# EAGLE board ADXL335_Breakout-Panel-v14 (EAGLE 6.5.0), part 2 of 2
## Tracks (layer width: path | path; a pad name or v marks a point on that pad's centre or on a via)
GND  (via drill 0.51)
  Top 0.254: 19.05,16.26 18.8,16.51 | C2.2 18.29,9.56
  other vias: 13.59,17.02 13.21,19.56 16.89,17.91 17.5,7.82
  pour Bottom: 6.86,22.1 24.64,22.1 24.64,6.86 6.86,6.86
  pour Top: 6.86,6.86 24.64,6.86 24.64,22.1 6.86,22.1
GND1  (via drill 0.51)
  Top 0.254: 37.34,16.26 37.08,16.51 | C6.2 36.58,9.56
  other vias: 31.88,17.02 31.5,19.56 35.18,17.91 35.79,7.82
  pour Bottom: 25.15,22.1 42.93,22.1 42.93,6.86 25.15,6.86
  pour Top: 25.15,6.86 42.93,6.86 42.93,22.1 25.15,22.1
GND2  (via drill 0.51)
  Top 0.254: 55.63,16.26 55.37,16.51 | C10.2 54.86,9.56
  other vias: 50.16,17.02 49.78,19.56 53.47,17.91 54.08,7.82
  pour Bottom: 43.43,22.1 61.21,22.1 61.21,6.86 43.43,6.86
  pour Top: 43.43,6.86 61.21,6.86 61.21,22.1 43.43,22.1
GND3  (via drill 0.51)
  Top 0.254: 73.91,16.26 73.66,16.51 | C14.2 73.15,9.56
  other vias: 68.45,17.02 68.07,19.56 71.75,17.91 72.36,7.82
  pour Bottom: 61.72,22.1 79.5,22.1 79.5,6.86 61.72,6.86
  pour Top: 61.72,6.86 79.5,6.86 79.5,22.1 61.72,22.1
GND4  (via drill 0.51)
  Top 0.254: 92.2,16.26 91.95,16.51 | C18.2 91.44,9.56
  other vias: 86.74,17.02 86.36,19.56 90.04,17.91 90.65,7.82
  pour Bottom: 80.01,22.1 97.79,22.1 97.79,6.86 80.01,6.86
  pour Top: 80.01,6.86 97.79,6.86 97.79,22.1 80.01,22.1
GND5  (via drill 0.51)
  Top 0.254: 110.49,16.26 110.24,16.51 | C22.2 109.73,9.56
  other vias: 105.03,17.02 104.65,19.56 108.33,17.91 108.94,7.82
  pour Bottom: 98.3,22.1 116.08,22.1 116.08,6.86 98.3,6.86
  pour Top: 98.3,6.86 116.08,6.86 116.08,22.1 98.3,22.1
GND6  (via drill 0.51)
  Top 0.254: 19.05,32 18.8,32.26 | C26.2 18.29,25.31
  other vias: 13.59,32.77 13.21,35.31 16.89,33.66 17.5,23.57
  pour Bottom: 6.86,37.85 24.64,37.85 24.64,22.61 6.86,22.61
  pour Top: 6.86,22.61 24.64,22.61 24.64,37.85 6.86,37.85
GND7  (via drill 0.51)
  Top 0.254: 37.34,32 37.08,32.26 | C30.2 36.58,25.31
  other vias: 31.88,32.77 31.5,35.31 35.18,33.66 35.79,23.57
  pour Bottom: 25.15,37.85 42.93,37.85 42.93,22.61 25.15,22.61
  pour Top: 25.15,22.61 42.93,22.61 42.93,37.85 25.15,37.85
GND8  (via drill 0.51)
  Top 0.254: 55.63,32 55.37,32.26 | C34.2 54.86,25.31
  other vias: 50.16,32.77 49.78,35.31 53.47,33.66 54.08,23.57
  pour Bottom: 43.43,37.85 61.21,37.85 61.21,22.61 43.43,22.61
  pour Top: 43.43,22.61 61.21,22.61 61.21,37.85 43.43,37.85
GND9  (via drill 0.51)
  Top 0.254: 73.91,32 73.66,32.26 | C38.2 73.15,25.31
  other vias: 68.45,32.77 68.07,35.31 71.75,33.66 72.36,23.57
  pour Bottom: 61.72,37.85 79.5,37.85 79.5,22.61 61.72,22.61
  pour Top: 61.72,22.61 79.5,22.61 79.5,37.85 61.72,37.85
GND10  (via drill 0.51)
  Top 0.254: 92.2,32 91.95,32.26 | C42.2 91.44,25.31
  other vias: 86.74,32.77 86.36,35.31 90.04,33.66 90.65,23.57
  pour Bottom: 80.01,37.85 97.79,37.85 97.79,22.61 80.01,22.61
  pour Top: 80.01,22.61 97.79,22.61 97.79,37.85 80.01,37.85
GND11  (via drill 0.51)
  Top 0.254: 110.49,32 110.24,32.26 | C46.2 109.73,25.31
  other vias: 105.03,32.77 104.65,35.31 108.33,33.66 108.94,23.57
  pour Bottom: 98.3,37.85 116.08,37.85 116.08,22.61 98.3,22.61
  pour Top: 98.3,22.61 116.08,22.61 116.08,37.85 98.3,37.85
GND12  (via drill 0.51)
  Top 0.254: 19.05,47.75 18.8,48.01 | C50.2 18.29,41.06
  other vias: 13.59,48.51 13.21,51.05 16.89,49.4 17.5,39.32
  pour Bottom: 6.86,53.59 24.64,53.59 24.64,38.35 6.86,38.35
  pour Top: 6.86,38.35 24.64,38.35 24.64,53.59 6.86,53.59
GND13  (via drill 0.51)
  Top 0.254: 37.34,47.75 37.08,48.01 | C54.2 36.58,41.06
  other vias: 31.88,48.51 31.5,51.05 35.18,49.4 35.79,39.32
  pour Bottom: 25.15,53.59 42.93,53.59 42.93,38.35 25.15,38.35
  pour Top: 25.15,38.35 42.93,38.35 42.93,53.59 25.15,53.59
GND14  (via drill 0.51)
  Top 0.254: 55.63,47.75 55.37,48.01 | C58.2 54.86,41.06
  other vias: 50.16,48.51 49.78,51.05 53.47,49.4 54.08,39.32
  pour Bottom: 43.43,53.59 61.21,53.59 61.21,38.35 43.43,38.35
  pour Top: 43.43,38.35 61.21,38.35 61.21,53.59 43.43,53.59
GND15  (via drill 0.51)
  Top 0.254: 73.91,47.75 73.66,48.01 | C62.2 73.15,41.06
  other vias: 68.45,48.51 68.07,51.05 71.75,49.4 72.36,39.32
  pour Bottom: 61.72,53.59 79.5,53.59 79.5,38.35 61.72,38.35
  pour Top: 61.72,38.35 79.5,38.35 79.5,53.59 61.72,53.59
GND16  (via drill 0.51)
  Top 0.254: 92.2,47.75 91.95,48.01 | C66.2 91.44,41.06
  other vias: 86.74,48.51 86.36,51.05 90.04,49.4 90.65,39.32
  pour Bottom: 80.01,53.59 97.79,53.59 97.79,38.35 80.01,38.35
  pour Top: 80.01,38.35 97.79,38.35 97.79,53.59 80.01,53.59
GND17  (via drill 0.51)
  Top 0.254: 110.49,47.75 110.24,48.01 | C70.2 109.73,41.06
  other vias: 105.03,48.51 104.65,51.05 108.33,49.4 108.94,39.32
  pour Bottom: 98.3,53.59 116.08,53.59 116.08,38.35 98.3,38.35
  pour Top: 98.3,38.35 116.08,38.35 116.08,53.59 98.3,53.59
GND18  (via drill 0.51)
  Top 0.254: 19.05,63.5 18.8,63.75 | C74.2 18.29,56.81
  other vias: 13.59,64.26 13.21,66.8 16.89,65.15 17.5,55.07
  pour Bottom: 6.86,69.34 24.64,69.34 24.64,54.1 6.86,54.1
  pour Top: 6.86,54.1 24.64,54.1 24.64,69.34 6.86,69.34
GND19  (via drill 0.51)
  Top 0.254: 37.34,63.5 37.08,63.75 | C78.2 36.58,56.81
  other vias: 31.88,64.26 31.5,66.8 35.18,65.15 35.79,55.07
  pour Bottom: 25.15,69.34 42.93,69.34 42.93,54.1 25.15,54.1
  pour Top: 25.15,54.1 42.93,54.1 42.93,69.34 25.15,69.34
GND20  (via drill 0.51)
  Top 0.254: 55.63,63.5 55.37,63.75 | C82.2 54.86,56.81
  other vias: 50.16,64.26 49.78,66.8 53.47,65.15 54.08,55.07
  pour Bottom: 43.43,69.34 61.21,69.34 61.21,54.1 43.43,54.1
  pour Top: 43.43,54.1 61.21,54.1 61.21,69.34 43.43,69.34
GND21  (via drill 0.51)
  Top 0.254: 73.91,63.5 73.66,63.75 | C86.2 73.15,56.81
  other vias: 68.45,64.26 68.07,66.8 71.75,65.15 72.36,55.07
  pour Bottom: 61.72,69.34 79.5,69.34 79.5,54.1 61.72,54.1
  pour Top: 61.72,54.1 79.5,54.1 79.5,69.34 61.72,69.34
GND22  (via drill 0.51)
  Top 0.254: 92.2,63.5 91.95,63.75 | C90.2 91.44,56.81
  other vias: 86.74,64.26 86.36,66.8 90.04,65.15 90.65,55.07
  pour Bottom: 80.01,69.34 97.79,69.34 97.79,54.1 80.01,54.1
  pour Top: 80.01,54.1 97.79,54.1 97.79,69.34 80.01,69.34
GND23  (via drill 0.51)
  Top 0.254: 110.49,63.5 110.24,63.75 | C94.2 109.73,56.81
  other vias: 105.03,64.26 104.65,66.8 108.33,65.15 108.94,55.07
  pour Bottom: 98.3,69.34 116.08,69.34 116.08,54.1 98.3,54.1
  pour Top: 98.3,54.1 116.08,54.1 116.08,69.34 98.3,69.34
GND24  (via drill 0.51)
  Top 0.254: 19.05,79.25 18.8,79.5 | C98.2 18.29,72.56
  other vias: 13.59,80.01 13.21,82.55 16.89,80.9 17.5,70.82
  pour Bottom: 6.86,85.09 24.64,85.09 24.64,69.85 6.86,69.85
  pour Top: 6.86,69.85 24.64,69.85 24.64,85.09 6.86,85.09
GND25  (via drill 0.51)
  Top 0.254: 37.34,79.25 37.08,79.5 | C102.2 36.58,72.56
  other vias: 31.88,80.01 31.5,82.55 35.18,80.9 35.79,70.82
  pour Bottom: 25.15,85.09 42.93,85.09 42.93,69.85 25.15,69.85
  pour Top: 25.15,69.85 42.93,69.85 42.93,85.09 25.15,85.09
GND26  (via drill 0.51)
  Top 0.254: 55.63,79.25 55.37,79.5 | C106.2 54.86,72.56
  other vias: 50.16,80.01 49.78,82.55 53.47,80.9 54.08,70.82
  pour Bottom: 43.43,85.09 61.21,85.09 61.21,69.85 43.43,69.85
  pour Top: 43.43,69.85 61.21,69.85 61.21,85.09 43.43,85.09
GND27  (via drill 0.51)
  Top 0.254: 73.91,79.25 73.66,79.5 | C110.2 73.15,72.56
  other vias: 68.45,80.01 68.07,82.55 71.75,80.9 72.36,70.82
  pour Bottom: 61.72,85.09 79.5,85.09 79.5,69.85 61.72,69.85
  pour Top: 61.72,69.85 79.5,69.85 79.5,85.09 61.72,85.09
GND28  (via drill 0.51)
  Top 0.254: 92.2,79.25 91.95,79.5 | C114.2 91.44,72.56
  other vias: 86.74,80.01 86.36,82.55 90.04,80.9 90.65,70.82
  pour Bottom: 80.01,85.09 97.79,85.09 97.79,69.85 80.01,69.85
  pour Top: 80.01,69.85 97.79,69.85 97.79,85.09 80.01,85.09
GND29  (via drill 0.51)
  Top 0.254: 110.49,79.25 110.24,79.5 | C118.2 109.73,72.56
  other vias: 105.03,80.01 104.65,82.55 108.33,80.9 108.94,70.82
  pour Bottom: 98.3,85.09 116.08,85.09 116.08,69.85 98.3,69.85
  pour Top: 98.3,69.85 116.08,69.85 116.08,85.09 98.3,85.09
GND30  (via drill 0.51)
  Top 0.254: 19.05,95 18.8,95.25 | C122.2 18.29,88.3
  other vias: 13.59,95.76 13.21,98.3 16.89,96.65 17.5,86.56
  pour Bottom: 6.86,100.84 24.64,100.84 24.64,85.6 6.86,85.6
  pour Top: 6.86,85.6 24.64,85.6 24.64,100.84 6.86,100.84
GND31  (via drill 0.51)
  Top 0.254: 37.34,95 37.08,95.25 | C126.2 36.58,88.3
  other vias: 31.88,95.76 31.5,98.3 35.18,96.65 35.79,86.56
  pour Bottom: 25.15,100.84 42.93,100.84 42.93,85.6 25.15,85.6
  pour Top: 25.15,85.6 42.93,85.6 42.93,100.84 25.15,100.84
GND32  (via drill 0.51)
  Top 0.254: 55.63,95 55.37,95.25 | C130.2 54.86,88.3
  other vias: 50.16,95.76 49.78,98.3 53.47,96.65 54.08,86.56
  pour Bottom: 43.43,100.84 61.21,100.84 61.21,85.6 43.43,85.6
  pour Top: 43.43,85.6 61.21,85.6 61.21,100.84 43.43,100.84
GND33  (via drill 0.51)
  Top 0.254: 73.91,95 73.66,95.25 | C134.2 73.15,88.3
  other vias: 68.45,95.76 68.07,98.3 71.75,96.65 72.36,86.56
  pour Bottom: 61.72,100.84 79.5,100.84 79.5,85.6 61.72,85.6
  pour Top: 61.72,85.6 79.5,85.6 79.5,100.84 61.72,100.84
GND34  (via drill 0.51)
  Top 0.254: 92.2,95 91.95,95.25 | C138.2 91.44,88.3
  other vias: 86.74,95.76 86.36,98.3 90.04,96.65 90.65,86.56
  pour Bottom: 80.01,100.84 97.79,100.84 97.79,85.6 80.01,85.6
  pour Top: 80.01,85.6 97.79,85.6 97.79,100.84 80.01,100.84
GND35  (via drill 0.51)
  Top 0.254: 110.49,95 110.24,95.25 | C142.2 109.73,88.3
  other vias: 105.03,95.76 104.65,98.3 108.33,96.65 108.94,86.56
  pour Bottom: 98.3,100.84 116.08,100.84 116.08,85.6 98.3,85.6
  pour Top: 98.3,85.6 116.08,85.6 116.08,100.84 98.3,100.84
GND36  (via drill 0.51)
  Top 0.254: 19.05,110.74 18.8,111 | C146.2 18.29,104.05
  other vias: 13.59,111.51 13.21,114.05 16.89,112.39 17.5,102.31
  pour Bottom: 6.86,116.59 24.64,116.59 24.64,101.35 6.86,101.35
  pour Top: 6.86,101.35 24.64,101.35 24.64,116.59 6.86,116.59
GND37  (via drill 0.51)
  Top 0.254: 37.34,110.74 37.08,111 | C150.2 36.58,104.05
  other vias: 31.88,111.51 31.5,114.05 35.18,112.39 35.79,102.31
  pour Bottom: 25.15,116.59 42.93,116.59 42.93,101.35 25.15,101.35
  pour Top: 25.15,101.35 42.93,101.35 42.93,116.59 25.15,116.59
GND38  (via drill 0.51)
  Top 0.254: 55.63,110.74 55.37,111 | C154.2 54.86,104.05
  other vias: 50.16,111.51 49.78,114.05 53.47,112.39 54.08,102.31
  pour Bottom: 43.43,116.59 61.21,116.59 61.21,101.35 43.43,101.35
  pour Top: 43.43,101.35 61.21,101.35 61.21,116.59 43.43,116.59
GND39  (via drill 0.51)
  Top 0.254: 73.91,110.74 73.66,111 | C158.2 73.15,104.05
  other vias: 68.45,111.51 68.07,114.05 71.75,112.39 72.36,102.31
  pour Bottom: 61.72,116.59 79.5,116.59 79.5,101.35 61.72,101.35
  pour Top: 61.72,101.35 79.5,101.35 79.5,116.59 61.72,116.59
GND40  (via drill 0.51)
  Top 0.254: 92.2,110.74 91.95,111 | C162.2 91.44,104.05
  other vias: 86.74,111.51 86.36,114.05 90.04,112.39 90.65,102.31
  pour Bottom: 80.01,116.59 97.79,116.59 97.79,101.35 80.01,101.35
  pour Top: 80.01,101.35 97.79,101.35 97.79,116.59 80.01,116.59
GND41  (via drill 0.51)
  Top 0.254: 110.49,110.74 110.24,111 | C166.2 109.73,104.05
  other vias: 105.03,111.51 104.65,114.05 108.33,112.39 108.94,102.31
  pour Bottom: 98.3,116.59 116.08,116.59 116.08,101.35 98.3,101.35
  pour Top: 98.3,101.35 116.08,101.35 116.08,116.59 98.3,116.59
ST  (via drill 0.51)
  Top 0.254: U$4.2 18.39,14.1 v20.95,14.1
  Bottom 0.254: v20.95,14.1 13.59,14.1 11.94,15.75 11.94,19.56 10.67,20.83 SL1.1
ST1  (via drill 0.51)
  Top 0.254: U$10.2 36.68,14.1 v39.24,14.1
  Bottom 0.254: v39.24,14.1 31.88,14.1 30.23,15.75 30.23,19.56 28.96,20.83 SL2.1
ST2  (via drill 0.51)
  Top 0.254: U$17.2 54.97,14.1 v57.53,14.1
  Bottom 0.254: v57.53,14.1 50.16,14.1 48.51,15.75 48.51,19.56 47.24,20.83 SL3.1
ST3  (via drill 0.51)
  Top 0.254: U$24.2 73.26,14.1 v75.82,14.1
  Bottom 0.254: v75.82,14.1 68.45,14.1 66.8,15.75 66.8,19.56 65.53,20.83 SL4.1
ST4  (via drill 0.51)
  Top 0.254: U$31.2 91.54,14.1 v94.11,14.1
  Bottom 0.254: v94.11,14.1 86.74,14.1 85.09,15.75 85.09,19.56 83.82,20.83 SL5.1
ST5  (via drill 0.51)
  Top 0.254: U$38.2 109.83,14.1 v112.39,14.1
  Bottom 0.254: v112.39,14.1 105.03,14.1 103.38,15.75 103.38,19.56 102.11,20.83 SL6.1
ST6  (via drill 0.51)
  Top 0.254: U$45.2 18.39,29.84 v20.95,29.84
  Bottom 0.254: v20.95,29.84 13.59,29.84 11.94,31.5 11.94,35.31 10.67,36.58 SL7.1
ST7  (via drill 0.51)
  Top 0.254: U$52.2 36.68,29.84 v39.24,29.84
  Bottom 0.254: v39.24,29.84 31.88,29.84 30.23,31.5 30.23,35.31 28.96,36.58 SL8.1
ST8  (via drill 0.51)
  Top 0.254: U$59.2 54.97,29.84 v57.53,29.84
  Bottom 0.254: v57.53,29.84 50.16,29.84 48.51,31.5 48.51,35.31 47.24,36.58 SL9.1
ST9  (via drill 0.51)
  Top 0.254: U$66.2 73.26,29.84 v75.82,29.84
  Bottom 0.254: v75.82,29.84 68.45,29.84 66.8,31.5 66.8,35.31 65.53,36.58 SL10.1
ST10  (via drill 0.51)
  Top 0.254: U$73.2 91.54,29.84 v94.11,29.84
  Bottom 0.254: v94.11,29.84 86.74,29.84 85.09,31.5 85.09,35.31 83.82,36.58 SL11.1
ST11  (via drill 0.51)
  Top 0.254: U$80.2 109.83,29.84 v112.39,29.84
  Bottom 0.254: v112.39,29.84 105.03,29.84 103.38,31.5 103.38,35.31 102.11,36.58 SL12.1
ST12  (via drill 0.51)
  Top 0.254: U$87.2 18.39,45.59 v20.95,45.59
  Bottom 0.254: v20.95,45.59 13.59,45.59 11.94,47.24 11.94,51.05 10.67,52.32 SL13.1
ST13  (via drill 0.51)
  Top 0.254: U$94.2 36.68,45.59 v39.24,45.59
  Bottom 0.254: v39.24,45.59 31.88,45.59 30.23,47.24 30.23,51.05 28.96,52.32 SL14.1
ST14  (via drill 0.51)
  Top 0.254: U$101.2 54.97,45.59 v57.53,45.59
  Bottom 0.254: v57.53,45.59 50.16,45.59 48.51,47.24 48.51,51.05 47.24,52.32 SL15.1
ST15  (via drill 0.51)
  Top 0.254: U$108.2 73.26,45.59 v75.82,45.59
  Bottom 0.254: v75.82,45.59 68.45,45.59 66.8,47.24 66.8,51.05 65.53,52.32 SL16.1
ST16  (via drill 0.51)
  Top 0.254: U$115.2 91.54,45.59 v94.11,45.59
  Bottom 0.254: v94.11,45.59 86.74,45.59 85.09,47.24 85.09,51.05 83.82,52.32 SL17.1
ST17  (via drill 0.51)
  Top 0.254: U$122.2 109.83,45.59 v112.39,45.59
  Bottom 0.254: v112.39,45.59 105.03,45.59 103.38,47.24 103.38,51.05 102.11,52.32 SL18.1
ST18  (via drill 0.51)
  Top 0.254: U$129.2 18.39,61.34 v20.95,61.34
  Bottom 0.254: v20.95,61.34 13.59,61.34 11.94,62.99 11.94,66.8 10.67,68.07 SL19.1
ST19  (via drill 0.51)
  Top 0.254: U$136.2 36.68,61.34 v39.24,61.34
  Bottom 0.254: v39.24,61.34 31.88,61.34 30.23,62.99 30.23,66.8 28.96,68.07 SL20.1
ST20  (via drill 0.51)
  Top 0.254: U$143.2 54.97,61.34 v57.53,61.34
  Bottom 0.254: v57.53,61.34 50.16,61.34 48.51,62.99 48.51,66.8 47.24,68.07 SL21.1
ST21  (via drill 0.51)
  Top 0.254: U$150.2 73.26,61.34 v75.82,61.34
  Bottom 0.254: v75.82,61.34 68.45,61.34 66.8,62.99 66.8,66.8 65.53,68.07 SL22.1
ST22  (via drill 0.51)
  Top 0.254: U$157.2 91.54,61.34 v94.11,61.34
  Bottom 0.254: v94.11,61.34 86.74,61.34 85.09,62.99 85.09,66.8 83.82,68.07 SL23.1
ST23  (via drill 0.51)
  Top 0.254: U$164.2 109.83,61.34 v112.39,61.34
  Bottom 0.254: v112.39,61.34 105.03,61.34 103.38,62.99 103.38,66.8 102.11,68.07 SL24.1
ST24  (via drill 0.51)
  Top 0.254: U$171.2 18.39,77.09 v20.95,77.09
  Bottom 0.254: v20.95,77.09 13.59,77.09 11.94,78.74 11.94,82.55 10.67,83.82 SL25.1
ST25  (via drill 0.51)
  Top 0.254: U$178.2 36.68,77.09 v39.24,77.09
  Bottom 0.254: v39.24,77.09 31.88,77.09 30.23,78.74 30.23,82.55 28.96,83.82 SL26.1
ST26  (via drill 0.51)
  Top 0.254: U$185.2 54.97,77.09 v57.53,77.09
  Bottom 0.254: v57.53,77.09 50.16,77.09 48.51,78.74 48.51,82.55 47.24,83.82 SL27.1
ST27  (via drill 0.51)
  Top 0.254: U$192.2 73.26,77.09 v75.82,77.09
  Bottom 0.254: v75.82,77.09 68.45,77.09 66.8,78.74 66.8,82.55 65.53,83.82 SL28.1
ST28  (via drill 0.51)
  Top 0.254: U$199.2 91.54,77.09 v94.11,77.09
  Bottom 0.254: v94.11,77.09 86.74,77.09 85.09,78.74 85.09,82.55 83.82,83.82 SL29.1
ST29  (via drill 0.51)
  Top 0.254: U$206.2 109.83,77.09 v112.39,77.09
  Bottom 0.254: v112.39,77.09 105.03,77.09 103.38,78.74 103.38,82.55 102.11,83.82 SL30.1
ST30  (via drill 0.51)
  Top 0.254: U$213.2 18.39,92.84 v20.95,92.84
  Bottom 0.254: v20.95,92.84 13.59,92.84 11.94,94.49 11.94,98.3 10.67,99.57 SL31.1
ST31  (via drill 0.51)
  Top 0.254: U$220.2 36.68,92.84 v39.24,92.84
  Bottom 0.254: v39.24,92.84 31.88,92.84 30.23,94.49 30.23,98.3 28.96,99.57 SL32.1
ST32  (via drill 0.51)
  Top 0.254: U$227.2 54.97,92.84 v57.53,92.84
  Bottom 0.254: v57.53,92.84 50.16,92.84 48.51,94.49 48.51,98.3 47.24,99.57 SL33.1
ST33  (via drill 0.51)
  Top 0.254: U$234.2 73.26,92.84 v75.82,92.84
  Bottom 0.254: v75.82,92.84 68.45,92.84 66.8,94.49 66.8,98.3 65.53,99.57 SL34.1
ST34  (via drill 0.51)
  Top 0.254: U$241.2 91.54,92.84 v94.11,92.84
  Bottom 0.254: v94.11,92.84 86.74,92.84 85.09,94.49 85.09,98.3 83.82,99.57 SL35.1
ST35  (via drill 0.51)
  Top 0.254: U$248.2 109.83,92.84 v112.39,92.84
  Bottom 0.254: v112.39,92.84 105.03,92.84 103.38,94.49 103.38,98.3 102.11,99.57 SL36.1
ST36  (via drill 0.51)
  Top 0.254: U$255.2 18.39,108.58 v20.95,108.58
  Bottom 0.254: v20.95,108.58 13.59,108.58 11.94,110.24 11.94,114.05 10.67,115.32 SL37.1
ST37  (via drill 0.51)
  Top 0.254: U$262.2 36.68,108.58 v39.24,108.58
  Bottom 0.254: v39.24,108.58 31.88,108.58 30.23,110.24 30.23,114.05 28.96,115.32 SL38.1
ST38  (via drill 0.51)
  Top 0.254: U$269.2 54.97,108.58 v57.53,108.58
  Bottom 0.254: v57.53,108.58 50.16,108.58 48.51,110.24 48.51,114.05 47.24,115.32 SL39.1
ST39  (via drill 0.51)
  Top 0.254: U$276.2 73.26,108.58 v75.82,108.58
  Bottom 0.254: v75.82,108.58 68.45,108.58 66.8,110.24 66.8,114.05 65.53,115.32 SL40.1
ST40  (via drill 0.51)
  Top 0.254: U$283.2 91.54,108.58 v94.11,108.58
  Bottom 0.254: v94.11,108.58 86.74,108.58 85.09,110.24 85.09,114.05 83.82,115.32 SL41.1
ST41  (via drill 0.51)
  Top 0.254: U$290.2 109.83,108.58 v112.39,108.58
  Bottom 0.254: v112.39,108.58 105.03,108.58 103.38,110.24 103.38,114.05 102.11,115.32 SL42.1
VCC
  Top 0.254: U$4.14 16.18,11.63 16.51,11.3 | U$4.15 16.84,11.63 16.51,11.3 | SL1.6 15.15,8.13 C2.1 16.51,9.56 16.51,11.3
VCC1
  Top 0.254: U$10.14 34.47,11.63 34.8,11.3 | U$10.15 35.12,11.63 34.8,11.3 | SL2.6 33.44,8.13 C6.1 34.8,9.56 34.8,11.3
VCC2
  Top 0.254: U$17.14 52.76,11.63 53.09,11.3 | U$17.15 53.41,11.63 53.09,11.3 | SL3.6 51.73,8.13 C10.1 53.09,9.56 53.09,11.3
VCC3
  Top 0.254: U$24.14 71.05,11.63 71.37,11.3 | U$24.15 71.7,11.63 71.37,11.3 | SL4.6 70.02,8.13 C14.1 71.37,9.56 71.37,11.3
VCC4
  Top 0.254: U$31.14 89.34,11.63 89.66,11.3 | U$31.15 89.99,11.63 89.66,11.3 | SL5.6 88.3,8.13 C18.1 89.66,9.56 89.66,11.3
VCC5
  Top 0.254: U$38.14 107.62,11.63 107.95,11.3 | U$38.15 108.28,11.63 107.95,11.3 | SL6.6 106.59,8.13 C22.1 107.95,9.56 107.95,11.3
VCC6
  Top 0.254: U$45.14 16.18,27.38 16.51,27.05 | U$45.15 16.84,27.38 16.51,27.05 | SL7.6 15.15,23.88 C26.1 16.51,25.31 16.51,27.05
VCC7
  Top 0.254: U$52.14 34.47,27.38 34.8,27.05 | U$52.15 35.12,27.38 34.8,27.05 | SL8.6 33.44,23.88 C30.1 34.8,25.31 34.8,27.05
VCC8
  Top 0.254: U$59.14 52.76,27.38 53.09,27.05 | U$59.15 53.41,27.38 53.09,27.05 | SL9.6 51.73,23.88 C34.1 53.09,25.31 53.09,27.05
VCC9
  Top 0.254: U$66.14 71.05,27.38 71.37,27.05 | U$66.15 71.7,27.38 71.37,27.05 | SL10.6 70.02,23.88 C38.1 71.37,25.31 71.37,27.05
VCC10
  Top 0.254: U$73.14 89.34,27.38 89.66,27.05 | U$73.15 89.99,27.38 89.66,27.05 | SL11.6 88.3,23.88 C42.1 89.66,25.31 89.66,27.05
VCC11
  Top 0.254: U$80.14 107.62,27.38 107.95,27.05 | U$80.15 108.28,27.38 107.95,27.05 | SL12.6 106.59,23.88 C46.1 107.95,25.31 107.95,27.05
VCC12
  Top 0.254: U$87.14 16.18,43.12 16.51,42.8 | U$87.15 16.84,43.12 16.51,42.8 | SL13.6 15.15,39.62 C50.1 16.51,41.06 16.51,42.8
VCC13
  Top 0.254: U$94.14 34.47,43.12 34.8,42.8 | U$94.15 35.12,43.12 34.8,42.8 | SL14.6 33.44,39.62 C54.1 34.8,41.06 34.8,42.8
VCC14
  Top 0.254: U$101.14 52.76,43.12 53.09,42.8 | U$101.15 53.41,43.12 53.09,42.8 | SL15.6 51.73,39.62 C58.1 53.09,41.06 53.09,42.8
VCC15
  Top 0.254: U$108.14 71.05,43.12 71.37,42.8 | U$108.15 71.7,43.12 71.37,42.8 | SL16.6 70.02,39.62 C62.1 71.37,41.06 71.37,42.8
VCC16
  Top 0.254: U$115.14 89.34,43.12 89.66,42.8 | U$115.15 89.99,43.12 89.66,42.8 | SL17.6 88.3,39.62 C66.1 89.66,41.06 89.66,42.8
VCC17
  Top 0.254: U$122.14 107.62,43.12 107.95,42.8 | U$122.15 108.28,43.12 107.95,42.8 | SL18.6 106.59,39.62 C70.1 107.95,41.06 107.95,42.8
VCC18
  Top 0.254: U$129.14 16.18,58.87 16.51,58.55 | U$129.15 16.84,58.87 16.51,58.55 | SL19.6 15.15,55.37 C74.1 16.51,56.81 16.51,58.55
VCC19
  Top 0.254: U$136.14 34.47,58.87 34.8,58.55 | U$136.15 35.12,58.87 34.8,58.55 | SL20.6 33.44,55.37 C78.1 34.8,56.81 34.8,58.55
VCC20
  Top 0.254: U$143.14 52.76,58.87 53.09,58.55 | U$143.15 53.41,58.87 53.09,58.55 | SL21.6 51.73,55.37 C82.1 53.09,56.81 53.09,58.55
VCC21
  Top 0.254: U$150.14 71.05,58.87 71.37,58.55 | U$150.15 71.7,58.87 71.37,58.55 | SL22.6 70.02,55.37 C86.1 71.37,56.81 71.37,58.55
VCC22
  Top 0.254: U$157.14 89.34,58.87 89.66,58.55 | U$157.15 89.99,58.87 89.66,58.55 | SL23.6 88.3,55.37 C90.1 89.66,56.81 89.66,58.55
VCC23
  Top 0.254: U$164.14 107.62,58.87 107.95,58.55 | U$164.15 108.28,58.87 107.95,58.55 | SL24.6 106.59,55.37 C94.1 107.95,56.81 107.95,58.55
VCC24
  Top 0.254: U$171.14 16.18,74.62 16.51,74.3 | U$171.15 16.84,74.62 16.51,74.3 | SL25.6 15.15,71.12 C98.1 16.51,72.56 16.51,74.3
VCC25
  Top 0.254: U$178.14 34.47,74.62 34.8,74.3 | U$178.15 35.12,74.62 34.8,74.3 | SL26.6 33.44,71.12 C102.1 34.8,72.56 34.8,74.3
VCC26
  Top 0.254: U$185.14 52.76,74.62 53.09,74.3 | U$185.15 53.41,74.62 53.09,74.3 | SL27.6 51.73,71.12 C106.1 53.09,72.56 53.09,74.3
VCC27
  Top 0.254: U$192.14 71.05,74.62 71.37,74.3 | U$192.15 71.7,74.62 71.37,74.3 | SL28.6 70.02,71.12 C110.1 71.37,72.56 71.37,74.3
VCC28
  Top 0.254: U$199.14 89.34,74.62 89.66,74.3 | U$199.15 89.99,74.62 89.66,74.3 | SL29.6 88.3,71.12 C114.1 89.66,72.56 89.66,74.3
VCC29
  Top 0.254: U$206.14 107.62,74.62 107.95,74.3 | U$206.15 108.28,74.62 107.95,74.3 | SL30.6 106.59,71.12 C118.1 107.95,72.56 107.95,74.3
VCC30
  Top 0.254: U$213.14 16.18,90.37 16.51,90.04 | U$213.15 16.84,90.37 16.51,90.04 | SL31.6 15.15,86.87 C122.1 16.51,88.3 16.51,90.04
VCC31
  Top 0.254: U$220.14 34.47,90.37 34.8,90.04 | U$220.15 35.12,90.37 34.8,90.04 | SL32.6 33.44,86.87 C126.1 34.8,88.3 34.8,90.04
VCC32
  Top 0.254: U$227.14 52.76,90.37 53.09,90.04 | U$227.15 53.41,90.37 53.09,90.04 | SL33.6 51.73,86.87 C130.1 53.09,88.3 53.09,90.04
VCC33
  Top 0.254: U$234.14 71.05,90.37 71.37,90.04 | U$234.15 71.7,90.37 71.37,90.04 | SL34.6 70.02,86.87 C134.1 71.37,88.3 71.37,90.04
VCC34
  Top 0.254: U$241.14 89.34,90.37 89.66,90.04 | U$241.15 89.99,90.37 89.66,90.04 | SL35.6 88.3,86.87 C138.1 89.66,88.3 89.66,90.04
VCC35
  Top 0.254: U$248.14 107.62,90.37 107.95,90.04 | U$248.15 108.28,90.37 107.95,90.04 | SL36.6 106.59,86.87 C142.1 107.95,88.3 107.95,90.04
VCC36
  Top 0.254: U$255.14 16.18,106.12 16.51,105.79 | U$255.15 16.84,106.12 16.51,105.79 | SL37.6 15.15,102.62 C146.1 16.51,104.05 16.51,105.79
VCC37
  Top 0.254: U$262.14 34.47,106.12 34.8,105.79 | U$262.15 35.12,106.12 34.8,105.79 | SL38.6 33.44,102.62 C150.1 34.8,104.05 34.8,105.79
VCC38
  Top 0.254: U$269.14 52.76,106.12 53.09,105.79 | U$269.15 53.41,106.12 53.09,105.79 | SL39.6 51.73,102.62 C154.1 53.09,104.05 53.09,105.79
VCC39
  Top 0.254: U$276.14 71.05,106.12 71.37,105.79 | U$276.15 71.7,106.12 71.37,105.79 | SL40.6 70.02,102.62 C158.1 71.37,104.05 71.37,105.79
VCC40
  Top 0.254: U$283.14 89.34,106.12 89.66,105.79 | U$283.15 89.99,106.12 89.66,105.79 | SL41.6 88.3,102.62 C162.1 89.66,104.05 89.66,105.79
VCC41
  Top 0.254: U$290.14 107.62,106.12 107.95,105.79 | U$290.15 108.28,106.12 107.95,105.79 | SL42.6 106.59,102.62 C166.1 107.95,104.05 107.95,105.79
XOUT
  Top 0.254: U$4.12 12.24,13.5 C4.1 12.03,13.72 10.03,13.72 9.53,13.21 SL1.4
XOUT1
  Top 0.254: U$10.12 30.53,13.5 C8.1 30.31,13.72 28.32,13.72 27.81,13.21 SL2.4
XOUT2
  Top 0.254: U$17.12 48.81,13.5 C12.1 48.6,13.72 46.61,13.72 46.1,13.21 SL3.4
XOUT3
  Top 0.254: U$24.12 67.1,13.5 C16.1 66.89,13.72 64.9,13.72 64.39,13.21 SL4.4
XOUT4
  Top 0.254: U$31.12 85.39,13.5 C20.1 85.18,13.72 83.19,13.72 82.68,13.21 SL5.4
XOUT5
  Top 0.254: U$38.12 103.68,13.5 C24.1 103.47,13.72 101.47,13.72 100.97,13.21 SL6.4
XOUT6
  Top 0.254: U$45.12 12.24,29.25 C28.1 12.03,29.46 10.03,29.46 9.53,28.96 SL7.4
XOUT7
  Top 0.254: U$52.12 30.53,29.25 C32.1 30.31,29.46 28.32,29.46 27.81,28.96 SL8.4
XOUT8
  Top 0.254: U$59.12 48.81,29.25 C36.1 48.6,29.46 46.61,29.46 46.1,28.96 SL9.4
XOUT9
  Top 0.254: U$66.12 67.1,29.25 C40.1 66.89,29.46 64.9,29.46 64.39,28.96 SL10.4
XOUT10
  Top 0.254: U$73.12 85.39,29.25 C44.1 85.18,29.46 83.19,29.46 82.68,28.96 SL11.4
XOUT11
  Top 0.254: U$80.12 103.68,29.25 C48.1 103.47,29.46 101.47,29.46 100.97,28.96 SL12.4
XOUT12
  Top 0.254: U$87.12 12.24,45 C52.1 12.03,45.21 10.03,45.21 9.53,44.7 SL13.4
XOUT13
  Top 0.254: U$94.12 30.53,45 C56.1 30.31,45.21 28.32,45.21 27.81,44.7 SL14.4
XOUT14
  Top 0.254: U$101.12 48.81,45 C60.1 48.6,45.21 46.61,45.21 46.1,44.7 SL15.4
XOUT15
  Top 0.254: U$108.12 67.1,45 C64.1 66.89,45.21 64.9,45.21 64.39,44.7 SL16.4
XOUT16
  Top 0.254: U$115.12 85.39,45 C68.1 85.18,45.21 83.19,45.21 82.68,44.7 SL17.4
XOUT17
  Top 0.254: U$122.12 103.68,45 C72.1 103.47,45.21 101.47,45.21 100.97,44.7 SL18.4
XOUT18
  Top 0.254: U$129.12 12.24,60.75 C76.1 12.03,60.96 10.03,60.96 9.53,60.45 SL19.4
XOUT19
  Top 0.254: U$136.12 30.53,60.75 C80.1 30.31,60.96 28.32,60.96 27.81,60.45 SL20.4
XOUT20
  Top 0.254: U$143.12 48.81,60.75 C84.1 48.6,60.96 46.61,60.96 46.1,60.45 SL21.4
XOUT21
  Top 0.254: U$150.12 67.1,60.75 C88.1 66.89,60.96 64.9,60.96 64.39,60.45 SL22.4
XOUT22
  Top 0.254: U$157.12 85.39,60.75 C92.1 85.18,60.96 83.19,60.96 82.68,60.45 SL23.4
XOUT23
  Top 0.254: U$164.12 103.68,60.75 C96.1 103.47,60.96 101.47,60.96 100.97,60.45 SL24.4
XOUT24
  Top 0.254: U$171.12 12.24,76.5 C100.1 12.03,76.71 10.03,76.71 9.53,76.2 SL25.4
XOUT25
  Top 0.254: U$178.12 30.53,76.5 C104.1 30.31,76.71 28.32,76.71 27.81,76.2 SL26.4
XOUT26
  Top 0.254: U$185.12 48.81,76.5 C108.1 48.6,76.71 46.61,76.71 46.1,76.2 SL27.4
XOUT27
  Top 0.254: U$192.12 67.1,76.5 C112.1 66.89,76.71 64.9,76.71 64.39,76.2 SL28.4
XOUT28
  Top 0.254: U$199.12 85.39,76.5 C116.1 85.18,76.71 83.19,76.71 82.68,76.2 SL29.4
XOUT29
  Top 0.254: U$206.12 103.68,76.5 C120.1 103.47,76.71 101.47,76.71 100.97,76.2 SL30.4
XOUT30
  Top 0.254: U$213.12 12.24,92.24 C124.1 12.03,92.46 10.03,92.46 9.53,91.95 SL31.4
XOUT31
  Top 0.254: U$220.12 30.53,92.24 C128.1 30.31,92.46 28.32,92.46 27.81,91.95 SL32.4
XOUT32
  Top 0.254: U$227.12 48.81,92.24 C132.1 48.6,92.46 46.61,92.46 46.1,91.95 SL33.4
XOUT33
  Top 0.254: U$234.12 67.1,92.24 C136.1 66.89,92.46 64.9,92.46 64.39,91.95 SL34.4
XOUT34
  Top 0.254: U$241.12 85.39,92.24 C140.1 85.18,92.46 83.19,92.46 82.68,91.95 SL35.4
XOUT35
  Top 0.254: U$248.12 103.68,92.24 C144.1 103.47,92.46 101.47,92.46 100.97,91.95 SL36.4
XOUT36
  Top 0.254: U$255.12 12.24,107.99 C148.1 12.03,108.2 10.03,108.2 9.53,107.7 SL37.4
XOUT37
  Top 0.254: U$262.12 30.53,107.99 C152.1 30.31,108.2 28.32,108.2 27.81,107.7 SL38.4
XOUT38
  Top 0.254: U$269.12 48.81,107.99 C156.1 48.6,108.2 46.61,108.2 46.1,107.7 SL39.4
XOUT39
  Top 0.254: U$276.12 67.1,107.99 C160.1 66.89,108.2 64.9,108.2 64.39,107.7 SL40.4
XOUT40
  Top 0.254: U$283.12 85.39,107.99 C164.1 85.18,108.2 83.19,108.2 82.68,107.7 SL41.4
XOUT41
  Top 0.254: U$290.12 103.68,107.99 C168.1 103.47,108.2 101.47,108.2 100.97,107.7 SL42.4
YOUT
  Top 0.254: U$4.10 12.92,14.8 C3.1 11.98,15.75 SL1.3
YOUT1
  Top 0.254: U$10.10 31.21,14.8 C7.1 30.27,15.75 SL2.3
YOUT2
  Top 0.254: U$17.10 49.5,14.8 C11.1 48.55,15.75 SL3.3
YOUT3
  Top 0.254: U$24.10 67.79,14.8 C15.1 66.84,15.75 SL4.3
YOUT4
  Top 0.254: U$31.10 86.07,14.8 C19.1 85.13,15.75 SL5.3
YOUT5
  Top 0.254: U$38.10 104.36,14.8 C23.1 103.42,15.75 SL6.3
YOUT6
  Top 0.254: U$45.10 12.92,30.55 C27.1 11.98,31.5 SL7.3
YOUT7
  Top 0.254: U$52.10 31.21,30.55 C31.1 30.27,31.5 SL8.3
YOUT8
  Top 0.254: U$59.10 49.5,30.55 C35.1 48.55,31.5 SL9.3
YOUT9
  Top 0.254: U$66.10 67.79,30.55 C39.1 66.84,31.5 SL10.3
YOUT10
  Top 0.254: U$73.10 86.07,30.55 C43.1 85.13,31.5 SL11.3
YOUT11
  Top 0.254: U$80.10 104.36,30.55 C47.1 103.42,31.5 SL12.3
YOUT12
  Top 0.254: U$87.10 12.92,46.3 C51.1 11.98,47.24 SL13.3
YOUT13
  Top 0.254: U$94.10 31.21,46.3 C55.1 30.27,47.24 SL14.3
YOUT14
  Top 0.254: U$101.10 49.5,46.3 C59.1 48.55,47.24 SL15.3
YOUT15
  Top 0.254: U$108.10 67.79,46.3 C63.1 66.84,47.24 SL16.3
YOUT16
  Top 0.254: U$115.10 86.07,46.3 C67.1 85.13,47.24 SL17.3
YOUT17
  Top 0.254: U$122.10 104.36,46.3 C71.1 103.42,47.24 SL18.3
YOUT18
  Top 0.254: U$129.10 12.92,62.05 C75.1 11.98,62.99 SL19.3
YOUT19
  Top 0.254: U$136.10 31.21,62.05 C79.1 30.27,62.99 SL20.3
YOUT20
  Top 0.254: U$143.10 49.5,62.05 C83.1 48.55,62.99 SL21.3
YOUT21
  Top 0.254: U$150.10 67.79,62.05 C87.1 66.84,62.99 SL22.3
YOUT22
  Top 0.254: U$157.10 86.07,62.05 C91.1 85.13,62.99 SL23.3
YOUT23
  Top 0.254: U$164.10 104.36,62.05 C95.1 103.42,62.99 SL24.3
YOUT24
  Top 0.254: U$171.10 12.92,77.8 C99.1 11.98,78.74 SL25.3
YOUT25
  Top 0.254: U$178.10 31.21,77.8 C103.1 30.27,78.74 SL26.3
YOUT26
  Top 0.254: U$185.10 49.5,77.8 C107.1 48.55,78.74 SL27.3
YOUT27
  Top 0.254: U$192.10 67.79,77.8 C111.1 66.84,78.74 SL28.3
YOUT28
  Top 0.254: U$199.10 86.07,77.8 C115.1 85.13,78.74 SL29.3
YOUT29
  Top 0.254: U$206.10 104.36,77.8 C119.1 103.42,78.74 SL30.3
YOUT30
  Top 0.254: U$213.10 12.92,93.54 C123.1 11.98,94.49 SL31.3
YOUT31
  Top 0.254: U$220.10 31.21,93.54 C127.1 30.27,94.49 SL32.3
YOUT32
  Top 0.254: U$227.10 49.5,93.54 C131.1 48.55,94.49 SL33.3
YOUT33
  Top 0.254: U$234.10 67.79,93.54 C135.1 66.84,94.49 SL34.3
YOUT34
  Top 0.254: U$241.10 86.07,93.54 C139.1 85.13,94.49 SL35.3
YOUT35
  Top 0.254: U$248.10 104.36,93.54 C143.1 103.42,94.49 SL36.3
YOUT36
  Top 0.254: U$255.10 12.92,109.29 C147.1 11.98,110.24 SL37.3
YOUT37
  Top 0.254: U$262.10 31.21,109.29 C151.1 30.27,110.24 SL38.3
YOUT38
  Top 0.254: U$269.10 49.5,109.29 C155.1 48.55,110.24 SL39.3
YOUT39
  Top 0.254: U$276.10 67.79,109.29 C159.1 66.84,110.24 SL40.3
YOUT40
  Top 0.254: U$283.10 86.07,109.29 C163.1 85.13,110.24 SL41.3
YOUT41
  Top 0.254: U$290.10 104.36,109.29 C167.1 103.42,110.24 SL42.3
ZOUT
  Top 0.254: SL1.2 13.46,18.29 14.48,19.3 C1.2 15.56,19.2 U$4.8
ZOUT1
  Top 0.254: SL2.2 31.75,18.29 32.77,19.3 C5.2 33.85,19.2 U$10.8
ZOUT2
  Top 0.254: SL3.2 50.04,18.29 51.05,19.3 C9.2 52.14,19.2 U$17.8
ZOUT3
  Top 0.254: SL4.2 68.33,18.29 69.34,19.3 C13.2 70.42,19.2 U$24.8
ZOUT4
  Top 0.254: SL5.2 86.61,18.29 87.63,19.3 C17.2 88.71,19.2 U$31.8
ZOUT5
  Top 0.254: SL6.2 104.9,18.29 105.92,19.3 C21.2 107,19.2 U$38.8
ZOUT6
  Top 0.254: SL7.2 13.46,34.04 14.48,35.05 C25.2 15.56,34.95 U$45.8
ZOUT7
  Top 0.254: SL8.2 31.75,34.04 32.77,35.05 C29.2 33.85,34.95 U$52.8
ZOUT8
  Top 0.254: SL9.2 50.04,34.04 51.05,35.05 C33.2 52.14,34.95 U$59.8
ZOUT9
  Top 0.254: SL10.2 68.33,34.04 69.34,35.05 C37.2 70.42,34.95 U$66.8
ZOUT10
  Top 0.254: SL11.2 86.61,34.04 87.63,35.05 C41.2 88.71,34.95 U$73.8
ZOUT11
  Top 0.254: SL12.2 104.9,34.04 105.92,35.05 C45.2 107,34.95 U$80.8
ZOUT12
  Top 0.254: SL13.2 13.46,49.78 14.48,50.8 C49.2 15.56,50.7 U$87.8
ZOUT13
  Top 0.254: SL14.2 31.75,49.78 32.77,50.8 C53.2 33.85,50.7 U$94.8
ZOUT14
  Top 0.254: SL15.2 50.04,49.78 51.05,50.8 C57.2 52.14,50.7 U$101.8
ZOUT15
  Top 0.254: SL16.2 68.33,49.78 69.34,50.8 C61.2 70.42,50.7 U$108.8
ZOUT16
  Top 0.254: SL17.2 86.61,49.78 87.63,50.8 C65.2 88.71,50.7 U$115.8
ZOUT17
  Top 0.254: SL18.2 104.9,49.78 105.92,50.8 C69.2 107,50.7 U$122.8
ZOUT18
  Top 0.254: SL19.2 13.46,65.53 14.48,66.55 C73.2 15.56,66.45 U$129.8
ZOUT19
  Top 0.254: SL20.2 31.75,65.53 32.77,66.55 C77.2 33.85,66.45 U$136.8
ZOUT20
  Top 0.254: SL21.2 50.04,65.53 51.05,66.55 C81.2 52.14,66.45 U$143.8
ZOUT21
  Top 0.254: SL22.2 68.33,65.53 69.34,66.55 C85.2 70.42,66.45 U$150.8
ZOUT22
  Top 0.254: SL23.2 86.61,65.53 87.63,66.55 C89.2 88.71,66.45 U$157.8
ZOUT23
  Top 0.254: SL24.2 104.9,65.53 105.92,66.55 C93.2 107,66.45 U$164.8
ZOUT24
  Top 0.254: SL25.2 13.46,81.28 14.48,82.3 C97.2 15.56,82.2 U$171.8
ZOUT25
  Top 0.254: SL26.2 31.75,81.28 32.77,82.3 C101.2 33.85,82.2 U$178.8
ZOUT26
  Top 0.254: SL27.2 50.04,81.28 51.05,82.3 C105.2 52.14,82.2 U$185.8
ZOUT27
  Top 0.254: SL28.2 68.33,81.28 69.34,82.3 C109.2 70.42,82.2 U$192.8
ZOUT28
  Top 0.254: SL29.2 86.61,81.28 87.63,82.3 C113.2 88.71,82.2 U$199.8
ZOUT29
  Top 0.254: SL30.2 104.9,81.28 105.92,82.3 C117.2 107,82.2 U$206.8
ZOUT30
  Top 0.254: SL31.2 13.46,97.03 14.48,98.04 C121.2 15.56,97.94 U$213.8
ZOUT31
  Top 0.254: SL32.2 31.75,97.03 32.77,98.04 C125.2 33.85,97.94 U$220.8
ZOUT32
  Top 0.254: SL33.2 50.04,97.03 51.05,98.04 C129.2 52.14,97.94 U$227.8
ZOUT33
  Top 0.254: SL34.2 68.33,97.03 69.34,98.04 C133.2 70.42,97.94 U$234.8
ZOUT34
  Top 0.254: SL35.2 86.61,97.03 87.63,98.04 C137.2 88.71,97.94 U$241.8
ZOUT35
  Top 0.254: SL36.2 104.9,97.03 105.92,98.04 C141.2 107,97.94 U$248.8
ZOUT36
  Top 0.254: SL37.2 13.46,112.78 14.48,113.79 C145.2 15.56,113.69 U$255.8
ZOUT37
  Top 0.254: SL38.2 31.75,112.78 32.77,113.79 C149.2 33.85,113.69 U$262.8
ZOUT38
  Top 0.254: SL39.2 50.04,112.78 51.05,113.79 C153.2 52.14,113.69 U$269.8
ZOUT39
  Top 0.254: SL40.2 68.33,112.78 69.34,113.79 C157.2 70.42,113.69 U$276.8
ZOUT40
  Top 0.254: SL41.2 86.61,112.78 87.63,113.79 C161.2 88.71,113.69 U$283.8
ZOUT41
  Top 0.254: SL42.2 104.9,112.78 105.92,113.79 C165.2 107,113.69 U$290.8

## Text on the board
Bottom: V14 | V14 | V14 | V14 | V14 | V14 | V14 | V14 | V14 | V14 | V14 | V14 | V14 | V14 | V14 | V14 | V14 | V14 | V14 | V14 | V14 | V14 | V14 | V14 | V14 | V14 | V14 | V14 | V14 | V14 | V14 | V14 | V14 | V14 | V14 | V14 | V14 | V14 | V14 | V14 | V14 | V14
tPlace: ADXL335 | ADXL335 | ADXL335 | ADXL335 | ADXL335 | ADXL335 | ST | ST | ST | ST | ST | ST | Z | Z | Z | Z | Z | Z | Y | X | Y | X | Y | X | Y | X | Y | X | Y | X | X | X | X | X | X | X | Y | Z | Y | Z | Y | Z | Y | Z | Y | Z | Y | Z | GND | GND | GND | GND | GND | GND | VCC | VCC | VCC | VCC | VCC | VCC | ADXL335 | ADXL335 | ADXL335 | ADXL335 | ADXL335 | ADXL335 | ST | ST | ST | ST | ST | ST | Z | Z | Z | Z | Z | Z | Y | X | Y | X | Y | X | Y | X | Y | X | Y | X | X | Y | X | Y | X | Y | X | Y | X | Y | X | Y | Z | Z | Z | Z | Z | Z | GND | GND | GND | GND | GND | GND | VCC | VCC | VCC | VCC | VCC | VCC | ADXL335 | ADXL335 | ADXL335 | ADXL335 | ADXL335 | ADXL335 | ST | ST | ST | ST | ST | ST | Z | Z | Z | Z | Z | Z | Y | X | Y | X | Y | X | Y | X | Y | X | Y | X | X | X | X | X | X | X | Y | Y | Y | Y | Y | Y | Z | Z | Z | Z | Z | Z | GND | GND | GND | GND | GND | GND | VCC | VCC | VCC | VCC | VCC | VCC | ADXL335 | ADXL335 | ADXL335 | ADXL335 | ADXL335 | ADXL335 | ST | ST | ST | ST | ST | ST | Z | Z | Z | Z | Z | Z | Y | X | Y | X | Y | X | Y | X | Y | X | Y | X | X | X | X | X | X | X | Y | Z | Y | Z | Y | Z | Y | Z | Y | Z | Y | Z | GND | GND | GND | GND | GND | GND | VCC | VCC | VCC | VCC | VCC | VCC | ADXL335 | ADXL335 | ADXL335 | ADXL335 | ADXL335 | ADXL335 | ST | ST | ST | ST | ST | ST | Z | Z | Z | Z | Z | Z | Y | X | Y | X | Y | X | Y | X | Y | X | Y | X | X | X | X | X | X | X | Y | Z | Y | Z | Y | Z | Y | Z | Y | Z | Y | Z | GND | GND | GND | GND | GND | GND | VCC | VCC | VCC | VCC | VCC | VCC | ADXL335 | ADXL335 | ADXL335 | ADXL335 | ADXL335 | ADXL335 | ST | ST | ST | ST | ST | ST | Z | Z | Z | Z | Z | Z | Y | X | Y | X | Y | X | Y | X | Y | X | Y | X | X | Y | X | Y | X | Y | X | Y | X | Y | X | Y | Z | Z | Z | Z | Z | Z | GND | GND | GND | GND | GND | GND | VCC | VCC | VCC | VCC | VCC | VCC | ADXL335 | ADXL335 | ADXL335 | ADXL335 | ADXL335 | ADXL335 | ST | ST | ST | ST | ST | ST | Z | Z | Z | Z | Z | Z | Y | X | Y | X | Y | X | Y | X | Y | X | Y | X | X | X | X | X | X | X | Y | Y | Y | Y | Y | Y | Z | Z | Z | Z | Z | Z | GND | GND | GND | GND | GND | GND | VCC | VCC | VCC | VCC | VCC | VCC
bPlace: Accelerometer | Accelerometer | Accelerometer | Accelerometer | Accelerometer | Accelerometer | Tri-Axis | Tri-Axis | Tri-Axis | Tri-Axis | Tri-Axis | Tri-Axis | Accelerometer | Accelerometer | Accelerometer | Accelerometer | Accelerometer | Accelerometer | Tri-Axis | Tri-Axis | Tri-Axis | Tri-Axis | Tri-Axis | Tri-Axis | Accelerometer | Accelerometer | Accelerometer | Accelerometer | Accelerometer | Accelerometer | Tri-Axis | Tri-Axis | Tri-Axis | Tri-Axis | Tri-Axis | Tri-Axis | Accelerometer | Accelerometer | Accelerometer | Accelerometer | Accelerometer | Accelerometer | Tri-Axis | Tri-Axis | Tri-Axis | Tri-Axis | Tri-Axis | Tri-Axis | Accelerometer | Accelerometer | Accelerometer | Accelerometer | Accelerometer | Accelerometer | Tri-Axis | Tri-Axis | Tri-Axis | Tri-Axis | Tri-Axis | Tri-Axis | Accelerometer | Accelerometer | Accelerometer | Accelerometer | Accelerometer | Accelerometer | Tri-Axis | Tri-Axis | Tri-Axis | Tri-Axis | Tri-Axis | Tri-Axis | Accelerometer | Accelerometer | Accelerometer | Accelerometer | Accelerometer | Accelerometer | Tri-Axis | Tri-Axis | Tri-Axis | Tri-Axis | Tri-Axis | Tri-Axis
